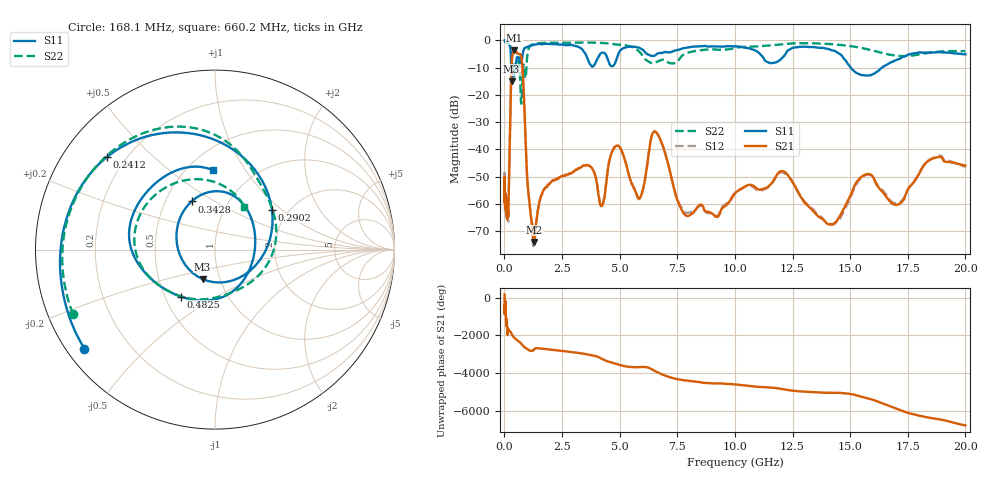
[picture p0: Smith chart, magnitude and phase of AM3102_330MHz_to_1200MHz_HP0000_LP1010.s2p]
! Date/Time: Tue, Sep 11, 2018 5:09 PM
! Network Analyzer: Agilent Technologies E8362B Rev: A.07.50.63
! Sweep from 0.010 to 20.000 GHz, 1601 Points, Sweep Type: LOG
! Power Supply: 4.950 V, 0.001 A
# Hz S DB R 50
!freq MagS11 AngS11 MagS21 AngS21 MagS12 AngS12 MagS22 AngS22
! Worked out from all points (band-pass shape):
!   1601 points, 10 MHz to 20 GHz, reference 50 ohm
!   highest |S21| = -3.59 dB at 438.8 MHz (marker M1); lowest = -74.0 dB at 1.302 GHz (marker M2)
!   |S21| within 3 dB of the highest: 329.8 MHz to 744.3 MHz (414.5 MHz wide, 77.2 % of centre)
!   lowest |S11| = -15.0 dB at 314.7 MHz (marker M3), VSWR 1.43, Z = 41.4 - j14 ohm
!   |S11| at or under -10 dB: 295.3 MHz to 348.7 MHz (53.38 MHz wide, 16.6 % of centre); 367.3 MHz to 479 MHz (111.8 MHz wide, 26.4 % of centre); 15.03 GHz to 16.38 GHz (1.355 GHz wide, 8.63 % of centre)
!   |S22| runs from -23.2 to -0.3 dB; largest |S21 - S12| = 0.012
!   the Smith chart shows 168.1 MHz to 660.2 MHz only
!   S11 on the Smith chart (normalised r, x): 168.1 MHz: 0.05, -0.34; 241.2 MHz: 0.13, +0.36; 290.2 MHz: 1.65, +0.86; 342.8 MHz: 0.67, +0.40; 482.5 MHz: 0.60, -0.35; 660.2 MHz: 0.66, +0.73
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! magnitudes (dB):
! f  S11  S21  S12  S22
! 10 MHz  0.0  -53.5  -55.2  -0.3
! 35.55 MHz  0.0  -56.9  -59.5  -0.5
! 126.4 MHz  -0.4  -63.1  -60.9  -1.0
! 168.1 MHz  -0.8  -63.2  -65.3  -1.2
! 241.2 MHz  -2.0  -34.7  -34.7  -1.8
! 290.2 MHz  -8.2  -14.3  -14.3  -3.6
! 314.7 MHz  -15.0  -8.3  -8.3  -6.0
! 342.8 MHz  -10.5  -5.8  -5.9  -8.1
! 438.8 MHz  -12.1  -3.6  -3.6  -11.0
! 447.2 MHz  -11.7  -3.6  -3.6  -10.6
! 482.5 MHz  -9.8  -3.7  -3.8  -9.0
! 660.2 MHz  -7.1  -5.0  -5.0  -10.8
! 1.302 GHz  -1.5  -74.0  -73.5  -1.2
! 1.59 GHz  -1.4  -57.1  -57.1  -0.9
! 4.23 GHz  -4.5  -60.8  -60.4  -0.9
! 4.878 GHz  -6.6  -38.6  -38.7  -1.5
! 5.652 GHz  -2.3  -54.8  -55.0  -2.9
! 6.58 GHz  -5.2  -33.7  -33.7  -8.0
! 7.958 GHz  -2.5  -64.5  -63.3  -4.5
! 12.09 GHz  -6.1  -48.1  -48.5  -1.3
! 14.14 GHz  -3.4  -67.5  -67.7  -1.3
! 20 GHz  -5.1  -46.0  -46.5  -3.9
